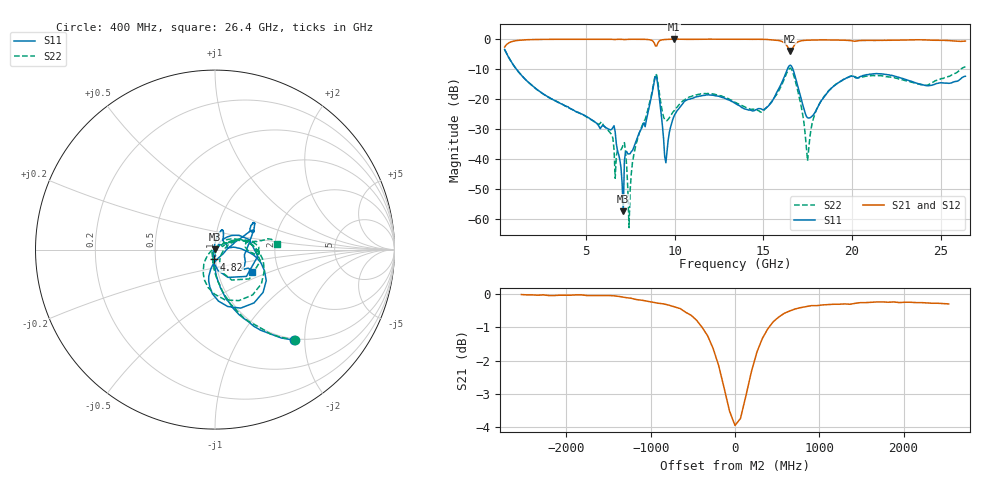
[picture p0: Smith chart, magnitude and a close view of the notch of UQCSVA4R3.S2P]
!  Part Number  UQCSVA4R3  Mounting Orientation: Horizontal
!  Description: Ultra Low ESR Microwave capacitors
!  Application: Coupling, Bypass, Tuning, DC Block
!  Filters, Matching
# GHZ S DB R 50
! Freq  |S11|  S11 Ph  |S21|  S21 Ph  |S12|  S12 Ph  |S22|  S22 Ph
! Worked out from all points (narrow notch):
!   401 points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, 400 MHz to 26.4 GHz, reference 50 ohm
!   highest |S21| = 0.02 dB at 9.955 GHz (marker M1); lowest = -3.9 dB at 16.52 GHz (marker M2)
!   notch at M2: 3.7 dB deep, 428 MHz wide at half that depth
!   lowest |S11| = -57.5 dB at 7.095 GHz (marker M3), VSWR 1.00, Z = 50 + j0.124 ohm
!   |S11| at or under -10 dB: 1.065 GHz to 16.36 GHz (15.29 GHz wide, 176 % of centre); 16.66 GHz to end of sweep
!   |S22| runs from -62.9 to -3.4 dB; largest |S21 - S12| = 0.012
!   S11 on the Smith chart (normalised r, x): 400 MHz: 0.97, -1.79; 4.82 GHz: 0.98, -0.11; 26.4 GHz: 1.45, -0.39
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0.4  -3.46 -48.7  -2.65 41.1  -2.66 41.0  -3.43 -48.3
1.375  -12.23 -79.4  -0.28 9.9  -0.29 9.9  -12.21 -79.1
4.755  -24.98 -96.4  -0.03 -13.0  -0.04 -13.1  -25.10 -103.9
4.82  -25.18 -96.5  -0.02 -13.3  -0.03 -13.4  -25.31 -104.5
6.51  -29.53 -89.8  -0.09 -21.4  -0.10 -21.5  -33.08 -136.6
7.095  -57.51 68.7  -0.10 -23.7  -0.11 -23.8  -35.20 -81.8
7.485  -38.22 5.8  -0.04 -25.0  -0.05 -25.1  -50.31 57.2
7.81  -34.09 33.9  -0.04 -26.8  -0.04 -26.9  -35.22 46.9
8.85  -13.98 16.0  -1.36 -37.5  -1.35 -37.4  -13.38 6.2
9.11  -18.55 -81.5  -0.71 -23.0  -0.73 -23.3  -17.13 -70.9
9.5  -41.27 153.3  -0.10 -29.1  -0.11 -29.2  -27.24 -29.6
9.955  -25.78 84.9  0.02 -32.5  0.00 -32.6  -23.98 12.6
11.255  -19.19 72.9  -0.05 -39.0  -0.07 -39.2  -18.60 22.9
13.4  -21.40 56.7  -0.04 -48.7  -0.06 -48.8  -21.07 26.2
15.155  -22.92 9.7  -0.09 -58.1  -0.11 -58.3  -23.02 42.2
16.52  -8.68 -53.8  -3.94 -60.4  -3.87 -60.5  -9.68 -50.3
17.04  -17.85 -102.8  -0.70 -52.2  -0.73 -52.4  -19.75 -127.3
17.43  -25.81 -70.8  -0.36 -57.2  -0.40 -57.3  -36.28 -179.9
17.755  -25.68 -23.6  -0.32 -59.5  -0.33 -59.7  -28.06 42.7
19.315  -14.21 26.5  -0.32 -68.6  -0.32 -68.9  -14.20 14.5
22.11  -11.95 29.8  -0.38 -81.0  -0.40 -81.3  -12.64 -6.3
26.4  -12.40 -31.6  -0.64 -102.8  -0.68 -103.3  -9.24 5.2
